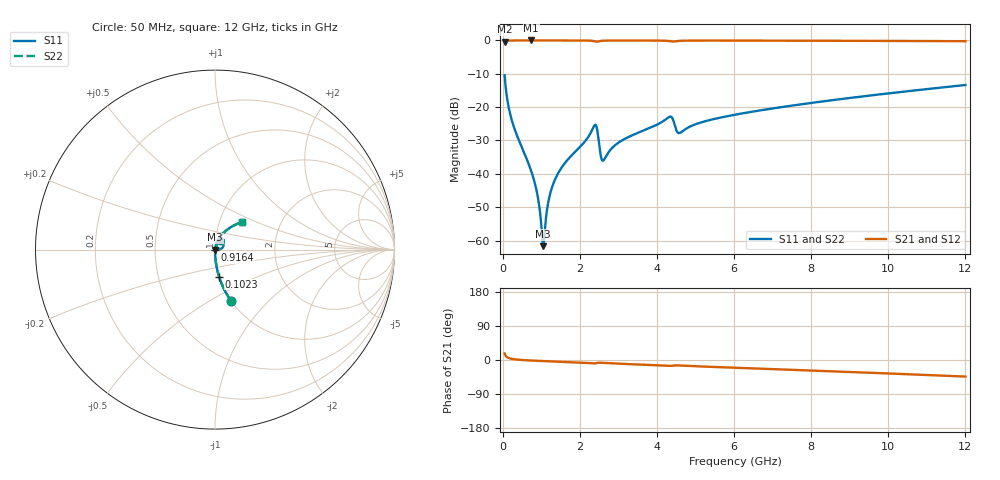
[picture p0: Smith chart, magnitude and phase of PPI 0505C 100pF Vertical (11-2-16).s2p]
# GHz S MA R 50
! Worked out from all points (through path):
!   1601 points, 50 MHz to 12 GHz, reference 50 ohm
!   highest |S21| = -0.01 dB at 737.1 MHz (marker M1); lowest = -0.4 dB at 50 MHz (marker M2)
!   group delay of S21, straight-line fit = 10.4 ps
!   lowest |S11| = -61.7 dB at 1.051 GHz (marker M3), VSWR 1.00, Z = 50.1 - j0.00794 ohm
!   |S11| at or under -10 dB: start of sweep to end of sweep
!   |S22| runs from -61.7 to -10.4 dB; largest |S21 - S12| = 0
!   S11 on the Smith chart (normalised r, x): 50 MHz: 1.00, -0.63; 102.3 MHz: 1.00, -0.31; 916.4 MHz: 1.00, -0.01; 12 GHz: 1.28, +0.41
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0.05  0.3018 -72.5  0.9531 17.4  0.9531 17.4  0.3018 -72.5
0.1022813  0.1519 -81.4  0.9881 8.5  0.9881 8.5  0.1519 -81.4
0.2740625  0.05396 -87.1  0.9981 2.4  0.9981 2.4  0.05396 -87.1
0.737125  0.01111 -87.7  0.9992 -1.3  0.9992 -1.3  0.01111 -87.7
0.916375  0.004329 -82.0  0.9992 -2.2  0.9992 -2.2  0.004329 -82.0
1.013469  0.001411 -57.8  0.9991 -2.7  0.9991 -2.7  0.001411 -57.8
1.050812  0.0008224 -5.5  0.9991 -2.8  0.9991 -2.8  0.0008224 -5.5
1.088156  0.001338 48.4  0.9991 -3.0  0.9991 -3.0  0.001338 48.4
1.207656  0.004417 75.0  0.999 -3.5  0.999 -3.5  0.004417 75.0
1.357031  0.00821 79.3  0.9989 -4.1  0.9989 -4.1  0.00821 79.3
2.044156  0.02676 78.4  0.9974 -7.0  0.9974 -7.0  0.02676 78.4
2.395188  0.05421 44.0  0.9662 -8.9  0.9662 -8.9  0.05421 44.0
2.5595  0.01705 23.8  0.9852 -7.4  0.9852 -7.4  0.01705 23.8
2.61925  0.01604 48.6  0.9909 -7.8  0.9909 -7.8  0.01604 48.6
3.0375  0.03022 75.3  0.9968 -9.9  0.9968 -9.9  0.03022 75.3
4.038312  0.05584 71.9  0.9941 -14.0  0.9941 -14.0  0.05584 71.9
4.352  0.07217 53.4  0.9714 -15.5  0.9714 -15.5  0.07217 53.4
4.591  0.04102 56.1  0.9853 -14.5  0.9853 -14.5  0.04102 56.1
6.025  0.07693 67.9  0.9944 -20.4  0.9944 -20.4  0.07693 67.9
8.019156  0.1159 61.0  0.9904 -27.9  0.9904 -27.9  0.1159 61.0
10.01331  0.1609 53.5  0.9837 -35.6  0.9837 -35.6  0.1609 53.5
12  0.2146 45.5  0.9729 -43.7  0.9729 -43.7  0.2146 45.5
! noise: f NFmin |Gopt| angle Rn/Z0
0.05  0.0003586  0.8538  0.3614  0.0005235
1.372  0.003677  0.6514  3.632  0.002003
2.701  0.01225  0.7784  7.196  0.01128
4.031  0.01277  0.6977  10.55  0.008186
5.36  0.01215  0.6024  13.79  0.005562
6.682  0.01268  0.5442  16.74  0.004852
8.012  0.0143  0.5238  19.72  0.005127
9.341  0.0161  0.513  22.64  0.005561
10.67  0.01803  0.5078  25.48  0.006082
12  0.02008  0.5068  28.26  0.006685
